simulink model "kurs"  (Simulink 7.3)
settings: Solver=ode45  StartTime=0.0  StopTime=40.0  RelTol=1e-3
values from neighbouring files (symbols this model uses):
  a_0 = 1    [kursach_ap_kren.m]
  a_0_sh = Tn*a_0    (= 1)    [kursach_ap_kren.m]
  a_1 = a1_shtrih+a4_shtrih+b1+myu_p*b3    [kursach_ap_kren.m]
  a_1_sh = a_0+Tn*a_1+myu_n*Tn*a3    [kursach_ap_kren.m]
  a_2 = b1*(a1_shtrih+a4_shtrih)+a2_shtrih+a1_shtrih*a4_shtrih+b2*b7+myu_p*b3*(a1_shtrih+a4_shtrih)+i_p*b3    [kursach_ap_kren.m]
  a_2_sh = a_1+Tn*a_2+myu_n*Tn*(a3*(a4_shtrih+b1+myu_p*b3)-a2_shtrih*a7)    [kursach_ap_kren.m]
  a_3 = b1*(a1_shtrih*a4_shtrih+a2_shtrih)+b2*b4+a1_shtrih*b2*b7+myu_p*b3*(a1_shtrih*a4_shtrih+a2_shtrih)+i_p*b3*(a1_shtrih+a4_shtrih)    [kursach_ap_kren.m]
  a_3_sh = a_2+Tn*a_3+myu_n*Tn*(a3*(a4_shtrih*b2+b2*b7)+i_p*a3*b3-myu_p*b3*(a2_shtrih*a7+a3*a4_shtrih)-a2_shtrih*a7*b1)    [kursach_ap_kren.m]
  a_4 = a1_shtrih*b2*b4+i_p*b3*(a1_shtrih*a4_shtrih+a2_shtrih)    [kursach_ap_kren.m]
  a_4_sh = a_3+Tn*a_4+myu_n*Tn*(a3*b2*b4-i_p*b3*(a2_shtrih*a7+a3*a4_shtrih))    [kursach_ap_kren.m]
  a_5_sh = a_4    [kursach_ap_kren.m]
  b4 = B(rezh,4)    [fash.m]    (also in kursach_ap_kren.m)
  b7 = B(rezh,6)    [fash.m]    (also in kursach_ap_kren.m)
  k = i_e_psi*i_p*b3*b4*a2_shtrih    [kursach_ap_kren.m]
  Tf1 = b7/b4    [kursach_ap_kren.m]
  Tn = 1    [kursach_ap_kren.m]

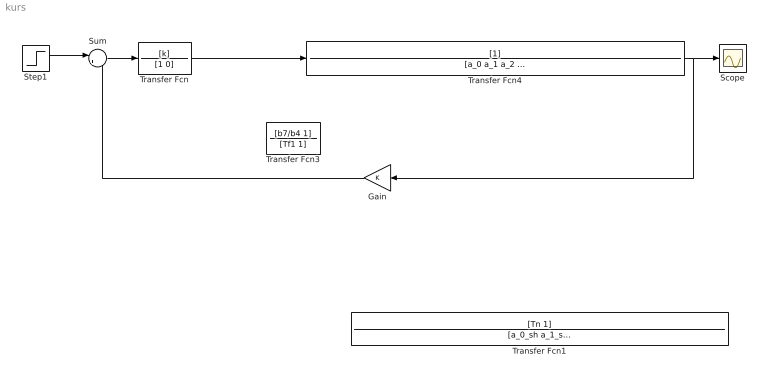
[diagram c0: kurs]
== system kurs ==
  Gain : Gain  ParameterDataType=fixdt(1, 16)  ParameterScaling=2^0  OutDataType=fixdt(1, 16)  OutScaling=2^0
  Scope : Scope
  Step1 : Step  Time=0  SampleTime=0
  Sum : Sum  Inputs=|+-  OutDataType=fixdt(1, 16)  OutScaling=2^0
  Transfer Fcn : TransferFcn  Numerator=[k]  Denominator=[1 0]
  Transfer Fcn1 : TransferFcn  Numerator=[Tn 1]  Denominator=[a_0_sh a_1_sh a_2_sh a_3_sh a_4_sh a_5_sh]
  Transfer Fcn3 : TransferFcn  Numerator=[b7/b4 1]  Denominator=[Tf1 1]
  Transfer Fcn4 : TransferFcn  Denominator=[a_0 a_1 a_2 a_3 a_4]
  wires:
  Transfer Fcn/1 -> Transfer Fcn4/1
  Transfer Fcn4/1 -> Scope/1, Gain/1
  Step1/1 -> Sum/1
  Sum/1 -> Transfer Fcn/1
  Gain/1 -> Sum/2
